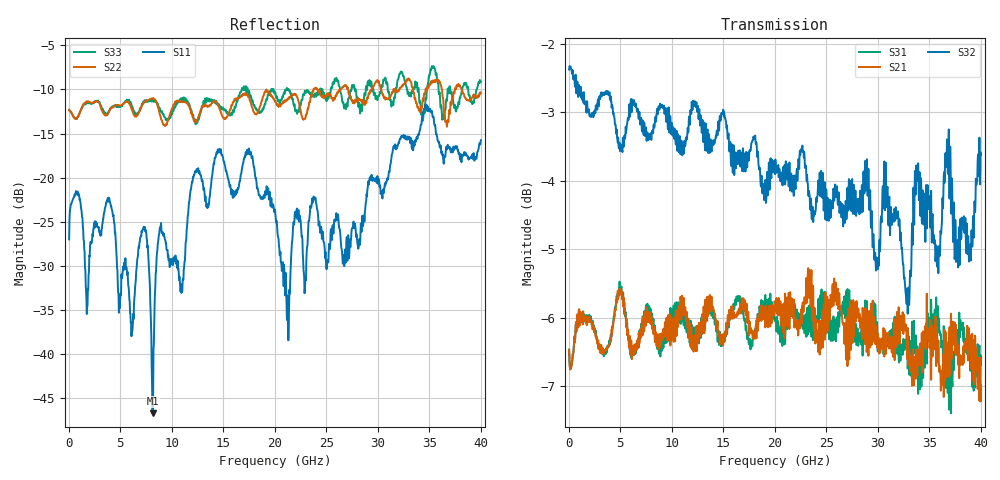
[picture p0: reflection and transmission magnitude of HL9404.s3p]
! 4/29/2021 8:38:01 AM
! H:\PRODUCTION_DATA\TEMP_S3P.S3P
! CHANNEL.1
! TR.MEASUREMENT
! CORRECTED.DATA
# GHZ S RI R 50.0
! FREQ.GHZ  S11RE  S11IM  S12RE  S12IM  S13RE  S13IM
!  S21RE  S21IM  S22RE  S22IM  S23RE  S23IM
!  S31RE  S31IM  S32RE  S32IM  S33RE  S33IM
!; PortSelection: Port_123
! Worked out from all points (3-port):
!   1143 points, 35 MHz to 40.01 GHz, reference 50 ohm
!   strongest paths, dB at 35 MHz, 10.01 GHz, 20.02 GHz, 30.03 GHz, 40.01 GHz:
!     S32: -2.4, -3.2, -3.9, -5.1, -3.6
!     S21: -6.5, -6.3, -5.8, -6.4, -7.0
!     S31: -6.5, -5.9, -6.0, -6.3, -6.7
!   lowest |S11| = -46.8 dB at 8.155 GHz (marker M1), VSWR 1.01, Z = 49.8 + j0.397 ohm
!   |S11| at or under -10 dB: start of sweep to end of sweep
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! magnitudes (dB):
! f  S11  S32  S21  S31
! 35 MHz  -27.0  -2.4  -6.5  -6.5
! 6.125 GHz  -36.9  -2.9  -6.6  -6.5
! 7.35 GHz  -25.7  -3.2  -6.1  -5.9
! 8.155 GHz  -46.8  -3.3  -6.1  -6.1
! 8.82 GHz  -25.9  -2.9  -6.4  -6.4
! 10.96 GHz  -32.1  -3.4  -5.9  -5.9
! 12.39 GHz  -19.1  -2.9  -6.4  -6.3
! 20.02 GHz  -23.6  -3.9  -5.8  -6.0
! 21.28 GHz  -35.2  -3.9  -6.0  -6.0
! 40.01 GHz  -15.8  -3.6  -7.0  -6.7
